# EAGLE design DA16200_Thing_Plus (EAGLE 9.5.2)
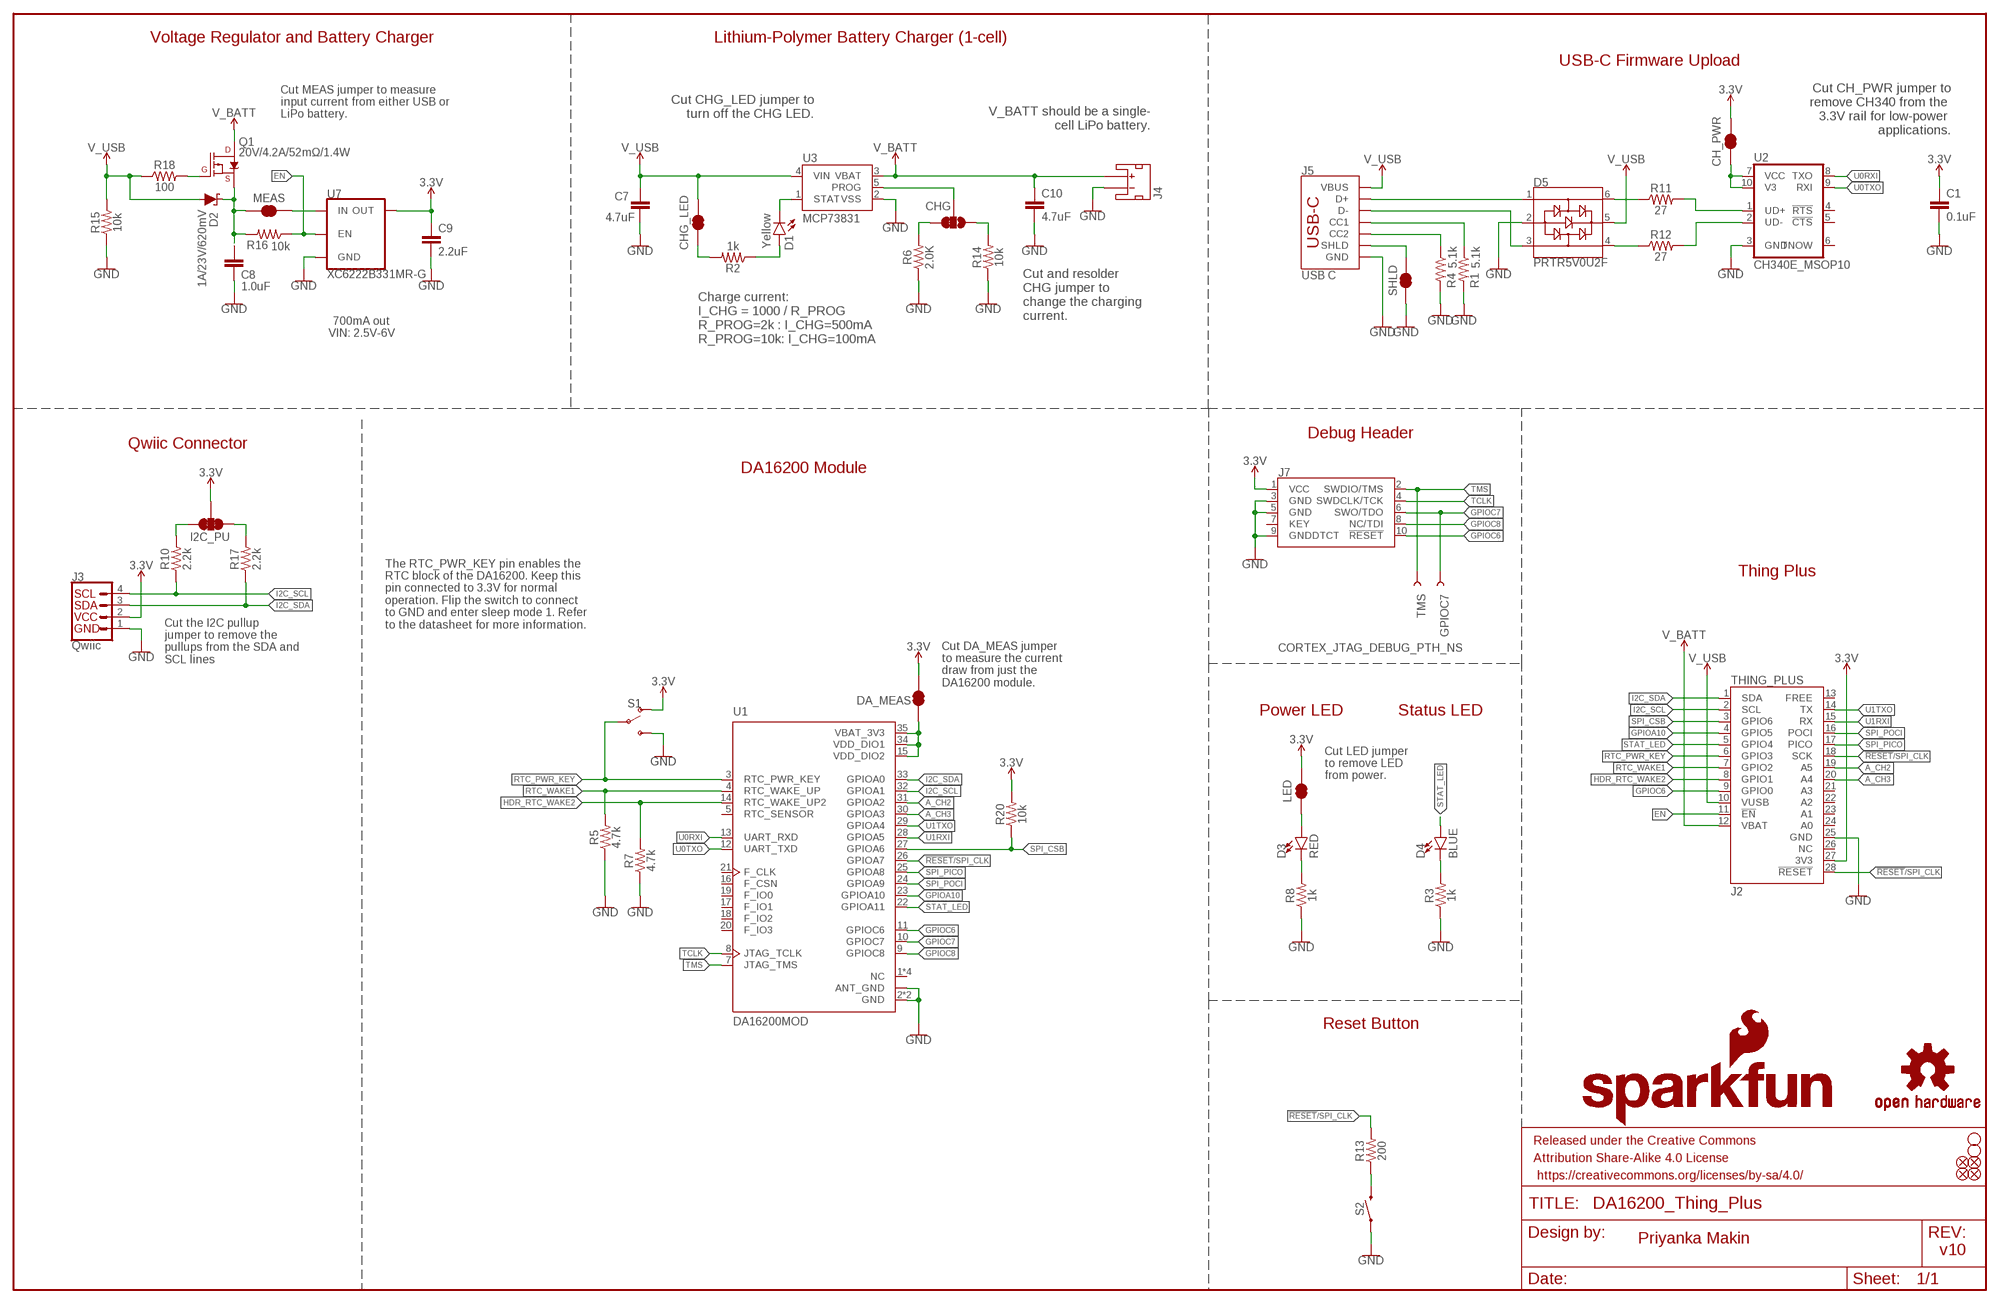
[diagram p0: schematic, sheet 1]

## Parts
C1  0.1uF  0.1UF-0402T-16V-10%  [0402-TIGHT]
C7  4.7uF  4.7UF-0402_TIGHT-6.3V-20%-X5R  [0402-TIGHT]
C8  1.0uF  1.0UF-0402T-16V-10%  [0402-TIGHT]
C9  2.2uF  2.2UF-0402_TIGHT-10V-10%-X5R  [0402-TIGHT]
C10  4.7uF  4.7UF-0402_TIGHT-6.3V-20%-X5R  [0402-TIGHT]
CH_PWR  JUMPER-SMT_2_NC_TRACE_SILK  [SMT-JUMPER_2_NC_TRACE_SILK]
CHG  JUMPER-SMT_3_1-NC_TRACE_SILK  [SMT-JUMPER_3_1-NC_TRACE_SILK]
CHG_LED  JUMPER-SMT_2_NC_TRACE_SILK  [SMT-JUMPER_2_NC_TRACE_SILK]
D1  Yellow  LED-YELLOW0603  [LED-0603]
D2  1A/23V/620mV  DIODE-SCHOTTKY-BAT20J  [SOD-323]
D3  RED  LED-RED0603  [LED-0603]
D4  BLUE  LED-BLUE0603  [LED-0603]
D5  PRTR5V0U2F  [SOT886]
DA_MEAS  JUMPER-SMT_2_NC_TRACE_SILK  [SMT-JUMPER_2_NC_TRACE_SILK]
FD1  FIDUCIALUFIDUCIAL  [FIDUCIAL-MICRO]
FD2  FIDUCIALUFIDUCIAL  [FIDUCIAL-MICRO]
FD3  FIDUCIALUFIDUCIAL  [FIDUCIAL-MICRO]
FD4  FIDUCIALUFIDUCIAL  [FIDUCIAL-MICRO]
FRAME1  FRAME-LEDGER  [CREATIVE_COMMONS]
GPIOC7  TEST-POINT3  [PAD.03X.03]
H3  STAND-OFF  [STAND-OFF]
H4  STAND-OFF  [STAND-OFF]
I2C_PU  JUMPER-SMT_3_2-NC_TRACE_SILK  [SMT-JUMPER_3_2-NC_TRACE_SILK]
J2  THING_PLUS  [THING_PLUS]
J3  Qwiic  QWIIC_CONNECTORJS-1MM  [JST04_1MM_RA]
J4  JST_2MM_MALE  [JST-2-SMD]
J5  USB C  USB_C_4-LAYER-ISOLATED  [USB-C-16P-4LAYER-ISOLATED]
J7  CORTEX_JTAG_DEBUG_PTH_NS  [2X5-PTH-1.27MM-NO_SILK]
LED  JUMPER-SMT_2_NC_TRACE_SILK  [SMT-JUMPER_2_NC_TRACE_SILK]
LOGO1  OSHW-LOGOS  [OSHW-LOGO-S]
LOGO2  SFE_LOGO_NAME_FLAME.1_INCH  [SFE_LOGO_NAME_FLAME_.1]
MEAS  JUMPER-COMBO_2_NC_TRACE  [COMBO-JUMPER_2_NC_TRACE]
Q1  20V/4.2A/52mΩ/1.4W  MOSFET_PCH-DMG2305UX-7  [SOT23-3]
R1  5.1k  5.1KOHM-0402T-1/16W-1%  [0402-TIGHT]
R2  1k  1KOHM-0402T-1/16W-1%  [0402-TIGHT]
R3  1k  1KOHM-0402T-1/16W-1%  [0402-TIGHT]
R4  5.1k  5.1KOHM-0402T-1/16W-1%  [0402-TIGHT]
R5  4.7k  4.7KOHM-0402T-1/16W-1%  [0402-TIGHT]
R6  2.0K  2.0KOHM-0402T-1/16W-1%  [0402-TIGHT]
R7  4.7k  4.7KOHM-0402T-1/16W-1%  [0402-TIGHT]
R8  1k  1KOHM-0402T-1/16W-1%  [0402-TIGHT]
R10  2.2k  2.2KOHM-0402T-1/16W-1%  [0402-TIGHT]
R11  27  27OHM  [0402-TIGHT]
R12  27  27OHM  [0402-TIGHT]
R13  200  200OHM-0402T-1/16W-1%  [0402-TIGHT]
R14  10k  10KOHM-0402T-1/16W-1%  [0402-TIGHT]
R15  10k  10KOHM-0402T-1/16W-1%  [0402-TIGHT]
R16  10k  10KOHM-0402T-1/16W-1%  [0402-TIGHT]
R17  2.2k  2.2KOHM-0402T-1/16W-1%  [0402-TIGHT]
R18  100  100OHM-0402-TIGHT-1/16W-1%  [0402-TIGHT]
R20  10k  10KOHM-0402T-1/16W-1%  [0402-TIGHT]
S1  SWITCH-SPDT-SMD-AYZ0202  [SWITCH_DPDT_SMD_AYZ0202]
S2  MOMENTARY-SWITCH-SPST-SMD-5.2MM-TALL  [TACTILE_SWITCH_SMD_5.2MM]
SHLD  JUMPER-SMT_2_NC_TRACE_SILK  [SMT-JUMPER_2_NC_TRACE_SILK]
TMS  TEST-POINT3  [PAD.03X.03]
U1  DA16200MOD  DA16200MOD-AAC4WA32  [XCVR_DA16200MOD-AAC4WA32]
U2  CH340E_MSOP10  [MSOP10]
U3  MCP73831  [SOT23-5]
U7  XC6222B331MR-G  [SOT23-5]

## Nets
3.3V: C1.1 C9.1 CH_PWR.2 DA_MEAS.2 I2C_PU.2 J2.27(3V3) J3.2 J7.1(VCC) LED.2 R20.2 S1.1(O) U7.5(OUT)
!RESET!/SPI_CLK: J2.18(SCK) J2.28(!RESET) R13.2 U1.26(GPIOA7)
A_CH2: J2.19(A5) U1.31(GPIOA2)
A_CH3: J2.20(A4) U1.30(GPIOA3)
EN: J2.11(!EN) R16.1 U7.3(EN)
GND: C1.2 C7.2 C8.2 C9.2 C10.2 D5.2 J2.25(GND) J3.1 J4.1(-) J5.GND J5.GND2(GND) J7.3(GND) J7.5(GND) J7.9(GNDDTCT) R1.2 R3.1 R4.2 R5.1 R6.1 R7.1 R8.1 R14.1 R15.1 S1.3(S) S2.1 SHLD.1 U1.2(GND) U1.ANT_GND U1.GND U2.3(GND) U3.2(VSS) U7.2(GND)
GPIOA10: J2.4(GPIO5) U1.23(GPIOA10)
GPIOC6: J2.9(GPIO0) J7.10(!RESET) U1.11(GPIOC6)
GPIOC7: GPIOC7.1 J7.6(SWO/TDO) U1.10(GPIOC7)
GPIOC8: J7.8(NC/TDI) U1.9(GPIOC8)
HDR_RTC_WAKE2: J2.8(GPIO1) R7.2 U1.14(RTC_WAKE_UP2)
I2C_SCL: J2.2(SCL) J3.4 R10.1 U1.32(GPIOA1)
I2C_SDA: J2.1(SDA) J3.3 R17.1 U1.33(GPIOA0)
N$1: D4.C R3.2
N$2: I2C_PU.3 R10.2
N$3: I2C_PU.1 R17.2
N$4: D3.A LED.1
N$5: D5.1 J5.A6(D+) J5.B6(D+)
N$6: D5.3 J5.A7(D-) J5.B7(D-)
N$7: D3.C R8.2
N$8: R13.1 S2.3
N$9: D1.C U3.1(STAT)
N$10: CHG.3 R6.2
N$11: J5.A5(CC1) R1.1
N$12: J5.B5(CC2) R4.1
N$13: D5.6 R11.1
N$14: CHG.2 U3.5(PROG)
N$15: C8.1 D2.C MEAS.1 MEAS.3 Q1.2(S) R16.2
N$16: D5.4 R12.1
N$17: D1.A R2.1
N$18: R11.2 U2.1(UD+)
N$19: R12.2 U2.2(UD-)
N$20: CHG.1 R14.2
N$21: Q1.1(G) R18.2
N$22: MEAS.2 MEAS.4 U7.1(IN)
N$23: CHG_LED.1 R2.2
N$24: J5.SHLD1(SHLD) J5.SHLD2(SHLD) J5.SHLD3(SHLD) J5.SHLD4(SHLD) J5.SHLD5(SHLD) J5.SHLD6(SHLD) J5.SHLD7(SHLD) J5.SHLD8(SHLD) SHLD.2
N$25: DA_MEAS.1 U1.15(VDD_DIO2) U1.34(VDD_DIO1) U1.35(VBAT_3V3)
N$26: CH_PWR.1 U2.7(VCC) U2.10(V3)
RTC_PWR_KEY: J2.6(GPIO3) S1.2(P) U1.3(RTC_PWR_KEY)
RTC_WAKE1: J2.7(GPIO2) R5.2 U1.4(RTC_WAKE_UP)
SPI_CSB: J2.3(GPIO6) R20.1 U1.27(GPIOA6)
SPI_PICO: J2.17(PICO) U1.25(GPIOA8)
SPI_POCI: J2.16(POCI) U1.24(GPIOA9)
STAT_LED: D4.A J2.5(GPIO4) U1.22(GPIOA11)
TCLK: J7.4(SWDCLK/TCK) U1.8(JTAG_TCLK)
TMS: J7.2(SWDIO/TMS) TMS.1 U1.7(JTAG_TMS)
U0RXI: U1.13(UART_RXD) U2.8(TXO)
U0TXO: U1.12(UART_TXD) U2.9(RXI)
U1RXI: J2.15(RX) U1.28(GPIOA5)
U1TXO: J2.14(TX) U1.29(GPIOA4)
V_BATT: C10.1 J2.12(VBAT) J4.2(+) Q1.3(D) U3.3(VBAT)
V_USB: C7.1 CHG_LED.2 D2.A D5.5 J2.10(VUSB) J5.VBUS1(VBUS) J5.VBUS2(VBUS) R15.2 R18.1 U3.4(VIN)
Unconnected: J2.13(FREE) J2.21(A3) J2.22(A2) J2.23(A1) J2.24(A0) J2.26(NC) J4.NC1(PAD1) J4.NC2(PAD2) J7.7(KEY) U1.1(NC) U1.5(RTC_SENSOR) U1.6(NC) U1.16(F_CSN) U1.17(F_IO1) U1.18(F_IO2) U1.19(F_IO0) U1.20(F_IO3) U1.21(F_CLK) U1.36(NC) U1.37(NC) U2.4(!RTS) U2.5(!CTS) U2.6(TNOW)

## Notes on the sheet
- Voltage Regulator and Battery Charger | Lithium-Polymer Battery Charger (1-cell)
- USB-C Firmware Upload
- Cut CH_PWR jumper to
  remove CH340 from the 
  3.3V rail for low-power 
  applications.
- Cut CHG_LED jumper to
  turn off the CHG LED.
- V_BATT should be a single-
  cell LiPo battery.
- Cut MEAS jumper to measure
  input current from either USB or 
  LiPo battery.
- Cut and resolder
  CHG jumper to 
  change the charging
  current.
- Charge current:
  I_CHG = 1000 / R_PROG
  R_PROG=2k : I_CHG=500mA
  R_PROG=10k: I_CHG=100mA
- 700mA out
  VIN: 2.5V-6V
- Debug Header
- Qwiic Connector
- DA16200 Module
- Thing Plus
- The RTC_PWR_KEY pin enables the 
  RTC block of the DA16200. Keep this 
  pin connected to 3.3V for normal 
  operation. Flip the switch to connect 
  to GND and enter sleep mode 1. Refer 
  to the datasheet for more information.
- Cut the I2C pullup 
  jumper to remove the 
  pullups from the SDA and 
  SCL lines
- Cut DA_MEAS jumper
  to measure the current
  draw from just the
  DA16200 module.
- Power LED | Status LED
- Cut LED jumper
  to remove LED
  from power.
- Reset Button
- Priyanka Makin
- v10

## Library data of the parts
C1 = SparkFun-Capacitors:0.1UF: 0.1µF ceramic capacitors; PROD_ID: CAP-12416
C7 C10 = SparkFun-Capacitors:4.7UF: 4.7µF ceramic capacitors; PROD_ID: CAP-14240
C8 = SparkFun-Capacitors:1.0UF: 1µF ceramic capacitors; PROD_ID: CAP-12417
C9 = SparkFun-Capacitors:2.2UF: 2.2µF ceramic capacitors; PROD_ID: CAP-14232
CH_PWR CHG_LED DA_MEAS LED SHLD = SparkFun-Jumpers:JUMPER-SMT_2_NC_TRACE: Normally closed trace jumper
CHG = SparkFun-Jumpers:JUMPER-SMT_3_1-NC_TRACE: Normally closed trace jumper (1 of 2 connections) This jumper has a trace between two pads so it's normally closed (NC). The other connection is normally open (NO). Use a razor knife to open the connection. For best results follow the IPC guidelines for cutting traces: Cutout at least 0.063 mm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
D1 = SparkFun-LED:LED-YELLOW: Yellow SMD LED; PROD_ID: DIO-09003
D2 = SparkFun-DiscreteSemi:DIODE-SCHOTTKY: Schottky diode; PROD_ID: DIO-11623
D3 = SparkFun-LED:LED-RED: Red SMD LED; PROD_ID: DIO-00819
D4 = SparkFun-LED:LED-BLUE: Blue SMD LED; PROD_ID: DIO-08575
D5 = SparkFun-IC-Power:PRTR5V0U2: A small ESD protection device. Most commonly used on USB D+/D- signals to protect large, expensive, or especially sensitive USB enabled devices.; PROD_ID: DIO-14084
FD1-FD4 = SparkFun-Aesthetics:FIDUCIAL: Fiducial Alignment Points
FRAME1 = SparkFun-Aesthetics:FRAME-LEDGER: Schematic Frame - Ledger
GPIOC7 TMS = SparkFun-Connectors:TEST-POINT: SparkFun Test Points
H3 H4 = SparkFun-Hardware:STAND-OFF: Stand Off
I2C_PU = SparkFun-Jumpers:JUMPER-SMT_3_2-NC_TRACE: Normally closed trace jumper (2 of 2 connections) This jumper has a trace between all three pads so they are normally closed (NC). Use a razor knife to open the connection(s). For best results follow the IPC guidelines for cutting traces: Cutout at least 0.063 mm (0.005 in). Remove all loose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
J2 = SparkFun-Boards:THING_PLUS
J3 = SparkFun-Connectors:QWIIC_CONNECTOR: SparkFun I2C Standard Qwiic Connector An SMD 1mm pitch JST connector makes it easy and quick (get it? Qwiic?) to connect I2C devices to each other. The Qwiic system enables fast and solderless connection between popular platforms and various sensors and actuators. We carry 200mm, 100mm, 50mm, and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; PROD_ID: CONN-13694; VALUE: QWIIC_RIGHT_ANGLE
J4 = SparkFun-Connectors:JST_2MM_MALE: JST 2MM MALE RA CONNECTOR Two pin, compact surface mount connector. Commonly used as a battery input connection point. We really like the solid locking feeling and high current rating on these small connectors. We use these all the time as battery connectors. Mates to single-cell LiPo batteries.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; PROD_ID: CONN-11443; SF_ID: PRT-08612
J5 = SparkFun-Connectors:USB_C: USB Type C 16Pin Connector Super Speed pins not available on the 16-pin purely SMD connector so this part is best for USB 2.0 implementations. D1 and D2 are tied together enabling D+/- no matter which way the cable is plugged into the connector. The two channel configuration pins (CC1/2) are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; PROD_ID: CONN-14122; VALUE: USB Female Type C Connector
J7 = SparkFun-Connectors:CORTEX_JTAG_DEBUG: Cortex Debug Connector - 10 pin Supports JTAG debug, Serial Wire debug, and Serial Wire Viewer. PTH and SMD connector options available. General Connector Information Products: PTH Connector -via Digi-Key SparkFun PSoc SparkFun T
LOGO1 = SparkFun-Aesthetics:OSHW-LOGO: Open-Source Hardware (OSHW) Logo
LOGO2 = SparkFun-Aesthetics:SFE_LOGO_NAME_FLAME: SparkFun Font Logo w/ Flame
MEAS = SparkFun-Jumpers:JUMPER-COMBO_2_NC_TRACE
Q1 = SparkFun-DiscreteSemi:MOSFET_PCH: P-channel MOSFETs Voltage controlled devices that allow control of high current outputs. SparkFun Products: SparkFun ESP32 Thing SparkFun ESP8266 Thing SparkFun Pi Servo HAT V2 DMG2305UX-7 (20V/4.2A/SOT23-3); PROD_ID: TRANS-14388
R1 R4 = SparkFun-Resistors:5.1KOHM; PROD_ID: RES-14340
R2 R3 R8 = SparkFun-Resistors:1KOHM: 1kΩ resistor; PROD_ID: RES-14342
R5 R7 = SparkFun-Resistors:4.7KOHM: 4.7kΩ resistor; PROD_ID: RES-15343
R6 = SparkFun-Resistors:2.0KOHM: 2kΩ resistor; PROD_ID: RES-15406
R10 R17 = SparkFun-Resistors:2.2KOHM: 2.2kΩ resistor; PROD_ID: RES-14341
R11 R12 = SparkFun-Resistors:27OHM: 27Ω resistor; PROD_ID: RES-15238
R13 = SparkFun-Resistors:200OHM: 200Ω resistor; PROD_ID: RES-15550
R14-R16 R20 = SparkFun-Resistors:10KOHM: 10kΩ resistor; PROD_ID: RES-14241
R18 = SparkFun-Resistors:100OHM: 100Ω resistor; PROD_ID: RES-14962
S1 = SparkFun-Switches:SWITCH-SPDT: Single Pole, Double Throw (SPDT) Switch Single-pole, double-throw (SPDT) switch. Variant Overview SMD-AYZ0202 Surface Mount DPDT Switch (COM-00597) Used on e.g. LilyPad Arduino USB - ATmega32U4 Board PTH-11.6X4.0MM SPDT Mini Power Switch (COM-00102) Used on e.g. SparkFun Simon Says - Through-Hole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; PROD_ID: SWCH-08179; SF_ID: COM-00597
S2 = SparkFun-Switches:MOMENTARY-SWITCH-SPST: Momentary Switch (Pushbutton) - SPST; PROD_ID: SWCH-14139
U1 = SparkFun-RF:DA16200MOD-AAC4WA32: Check prices; PROD_ID: IC-16179
U2 = SparkFun-IC-Comms:CH340E; PROD_ID: IC-14135
U3 = SparkFun-IC-Power:MCP73831: MCP73831T Li-Ion, Li-Pol Controller Miniature single cell, fully integrated Li-Ion, Li-polymer charge management controller Datasheet SparkFun Products: SparkFun ESP32 Thing SparkFun 9DoF Razor IMU M0; PROD_ID: IC-09995
U7 = SparkFun-IC-Power:XC6222; IOUT: 700mA; PROD_ID: VREG-16775; VOUT: 3.3V

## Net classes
0 default: width 0 mm, drill 0 mm
2 Clock: width 0.089 mm, clearance 0.178 mm

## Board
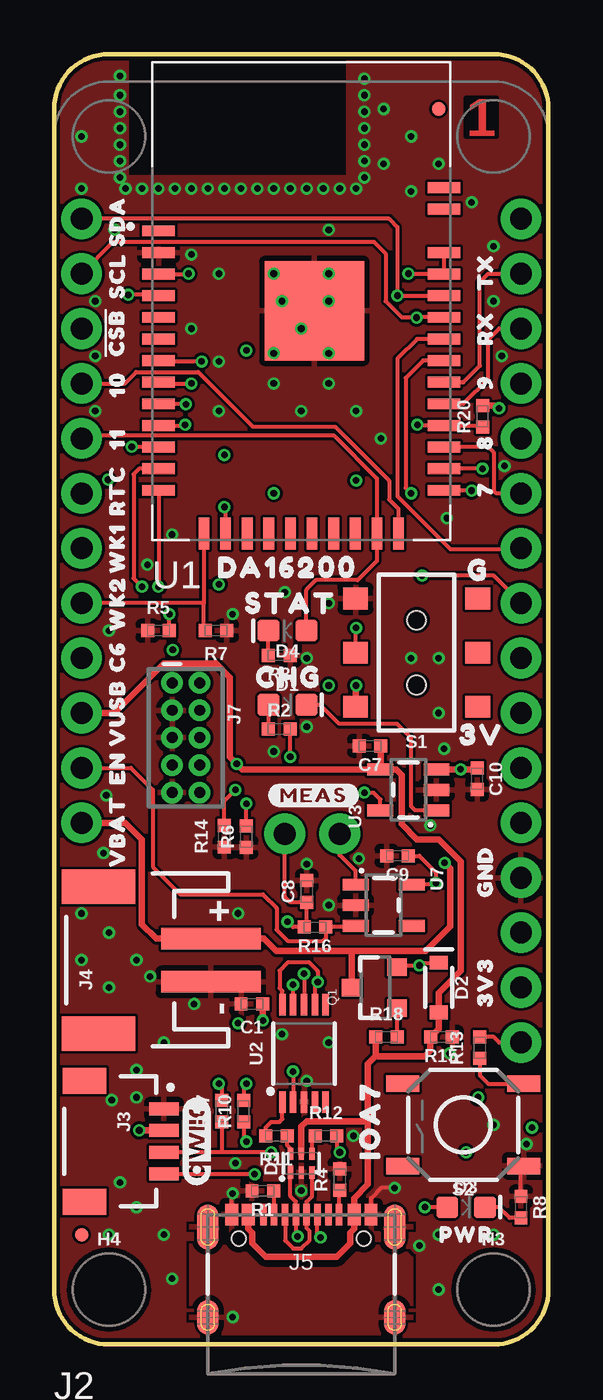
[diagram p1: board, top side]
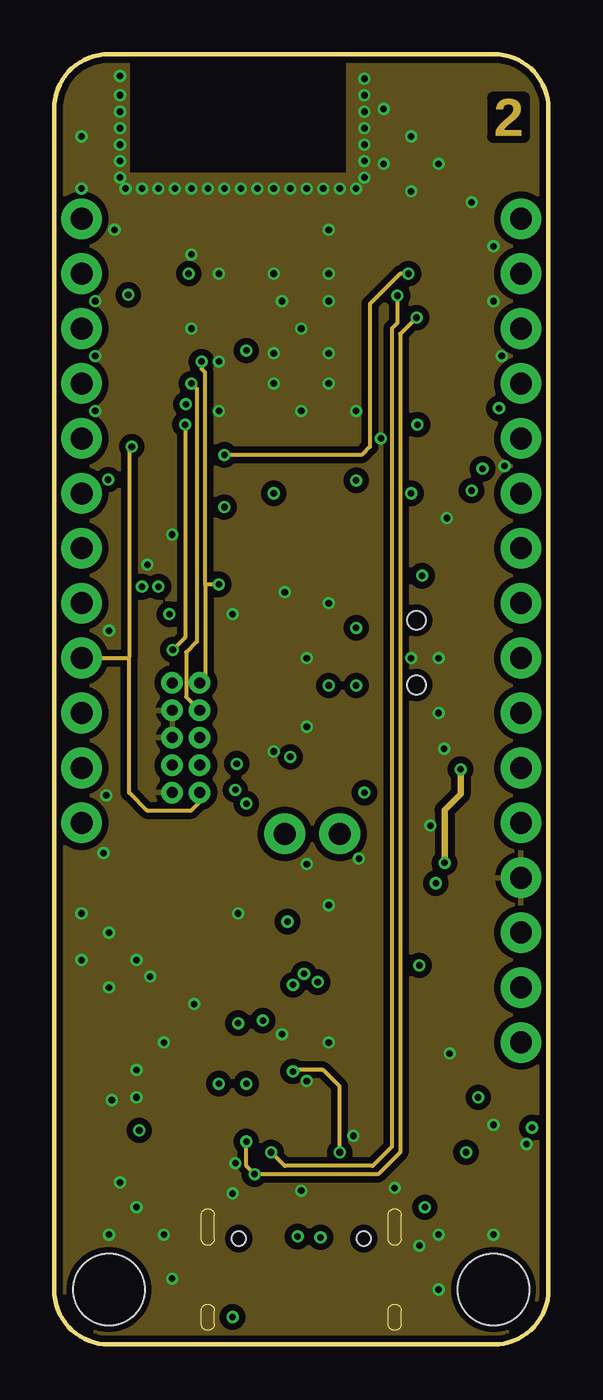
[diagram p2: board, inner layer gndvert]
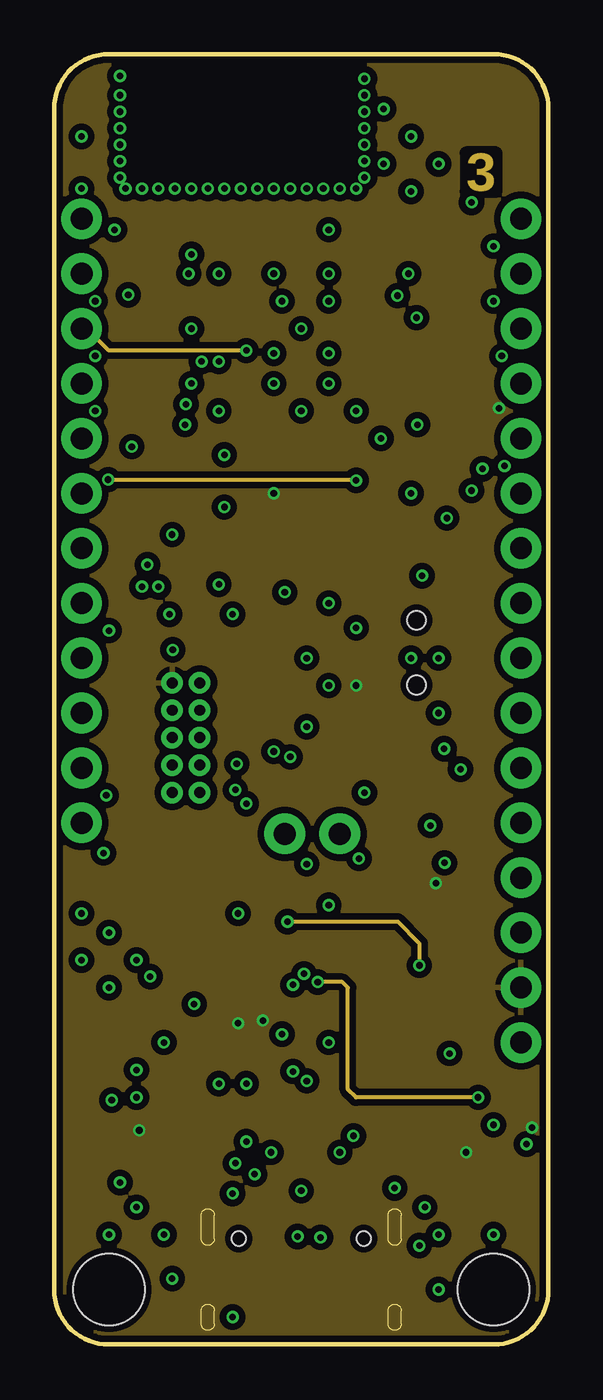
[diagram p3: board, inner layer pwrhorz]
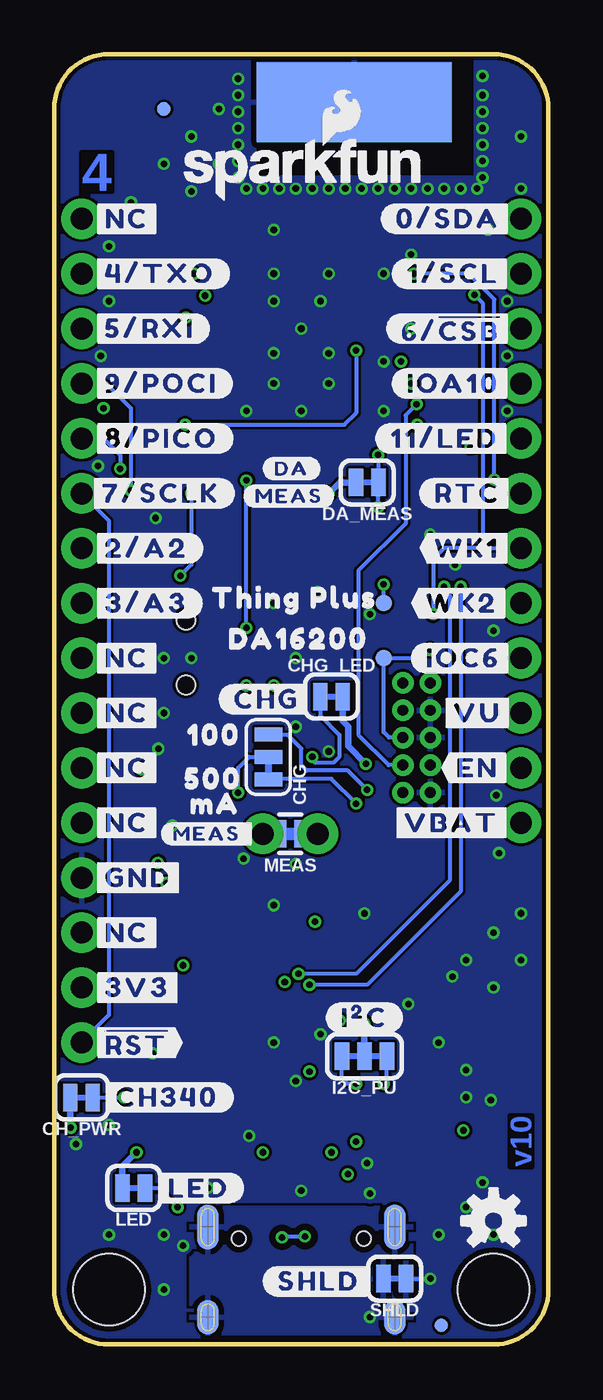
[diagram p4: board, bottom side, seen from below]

Size 22.86 x 59.69 mm. Coordinates in mm from the lower left corner, seen from the top.
Outline: 2.54,59.69 20.32,59.69 arc-90 22.86,57.15 22.86,2.54 arc-90 20.32,0 2.54,0 arc-90 0,2.54 0,57.15 arc-90 2.54,59.69
Copper layers (1*2*15*16): Top 0.035559375mm / dielectric 0.47751875mm / gndvert 0.035559375mm / dielectric 0.47751875mm / pwrhorz 0.035559375mm / dielectric 0.47751875mm / Bottom 0.035559375mm
Design rules "SparkFun-4-Layer-Minimum-JLCPCB": minimum track width 5mil, minimum drill 0.2mm, track to track 5mil, track to pad 5mil, pad to pad 5mil, via to via 5mil, smd to smd 5mil, copper to edge 7mil, drill to drill 7mil, minimum pad ring 5mil, minimum via ring 5mil, stop-mask expansion 2.5mil, vias tented up to drill 25mil, thermal gap 10mil

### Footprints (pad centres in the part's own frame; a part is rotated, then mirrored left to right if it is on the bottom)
0402-TIGHT = smd 0.6 x 0.6: 1 -0.5,0; 2 0.5,0
SMT-JUMPER_2_NC_TRACE_SILK = smd 0.66 x 1.27: 1 -0.521,0; 2 0.521,0
SMT-JUMPER_3_1-NC_TRACE_SILK = smd 0.66 x 1.27: 1 -1.041,0; 2 0,0; 3 1.041,0
LED-0603 = smd 1 x 1: A -0.877,0; C 0.877,0
SOD-323 = smd 0.63 x 0.83: A 1.15,0; C -1.15,0
SOT886 = smd 0.61 x 0.25: 1 -0.405,0.5 | smd 0.56 x 0.25: 2 -0.43,0; 3 -0.43,-0.5; 4 0.43,-0.5; 5 0.43,0; 6 0.43,0.5
FIDUCIAL-MICRO = smd 0.635 x 0.635: 1 0,0
PAD.03X.03 = smd 0.762 x 0.762: 1 0,0
STAND-OFF = hole 3.302: 0,0
SMT-JUMPER_3_2-NC_TRACE_SILK = smd 0.66 x 1.27: 1 -1.041,0; 2 0,0; 3 1.041,0
THING_PLUS = drill 1.016 pad 1.88: 1 1.27,52.07; 2 1.27,49.53; 3 1.27,46.99; 4 1.27,44.45; 5 1.27,41.91; 6 1.27,39.37; 7 1.27,36.83; 8 1.27,34.29; 9 1.27,31.75; 10 1.27,29.21; 11 1.27,26.67; 12 1.27,24.13; 13 21.59,52.07; 14 21.59,49.53; 15 21.59,46.99; 16 21.59,44.45; 17 21.59,41.91; 18 21.59,39.37; 19 21.59,36.83; 20 21.59,34.29; 21 21.59,31.75; 22 21.59,29.21; 23 21.59,26.67; 24 21.59,24.13; 25 21.59,21.59; 26 21.59,19.05; 27 21.59,16.51; 28 21.59,13.97
JST04_1MM_RA = smd 0.6 x 1.35: 1 -1.5,0; 2 -0.5,0; 3 0.5,0; 4 1.5,0 | smd 1.2 x 2: NC1 2.8,-3.675; NC2 -2.8,-3.675
JST-2-SMD = smd 1 x 4.6: 1 -1,-3.7; 2 1,-3.7 | smd 1.6 x 3.4: NC1 -3.4,1.5; NC2 3.4,1.5
USB-C-16P-4LAYER-ISOLATED = smd 0.3 x 1: A5 -1.25,-0.34; A6 -0.25,-0.34; A7 0.25,-0.34; A8 1.25,-0.34; B5 1.75,-0.34; B6 0.75,-0.34; B7 -0.75,-0.34; B8 -1.75,-0.34 | smd 0.6 x 1: GND -3.225,-0.34; GND2 3.225,-0.34; VBUS1 -2.45,-0.34; VBUS2 2.45,-0.34 | smd 1 x 2.1: SHLD1 -4.32,-0.915; SHLD2 4.32,-0.915 | smd 1 x 2.1 bottom: SHLD3 -4.32,-0.915; SHLD4 4.32,-0.915 | smd 1 x 1.6: SHLD5 -4.32,-5.095; SHLD8 4.32,-5.095 | smd 1 x 1.6 bottom: SHLD6 -4.32,-5.095; SHLD7 4.32,-5.095 | hole 0.65: -2.89,-1.445; 2.89,-1.445
2X5-PTH-1.27MM-NO_SILK = drill 0.508 pad 1: 1 -2.54,-0.635; 2 -2.54,0.635; 3 -1.27,-0.635; 4 -1.27,0.635; 5 0,-0.635; 6 0,0.635; 7 1.27,-0.635; 8 1.27,0.635; 9 2.54,-0.635; 10 2.54,0.635
COMBO-JUMPER_2_NC_TRACE = smd 0.635 x 1.27: 1 -0.508,0; 2 0.508,0 | drill 1.016 pad 1.88: 3 -1.27,0; 4 1.27,0
SOT23-3 = smd 0.8 x 0.9: 1 -0.95,-1; 2 0.95,-1; 3 0,1.1
SWITCH_DPDT_SMD_AYZ0202 = smd 1 x 1.15: 1 -2.5,2.825; 2 0,2.825; 3 2.5,2.825; 4 -2.5,-2.825; 5 0,-2.825; 6 2.5,-2.825 | hole 0.85: 1.5,0; -1.5,0
TACTILE_SWITCH_SMD_5.2MM = smd 1.524 x 0.762: 1 -2.794,1.905; 2 2.794,1.905; 3 -2.794,-1.905; 4 2.794,-1.905
XCVR_DA16200MOD-AAC4WA32 = smd 1.5 x 0.5: 1 -6.6,3.25; 2 -6.6,2.25; 3 -6.6,1.25; 4 -6.6,0.25; 5 -6.6,-0.75; 6 -6.6,-1.75; 7 -6.6,-2.75; 8 -6.6,-3.75; 9 -6.6,-4.75; 10 -6.6,-5.75; 11 -6.6,-6.75; 12 -6.6,-7.75; 13 -6.6,-8.75; 24 6.6,-8.75; 25 6.6,-7.75; 26 6.6,-6.75; 27 6.6,-5.75; 28 6.6,-4.75; 29 6.6,-3.75; 30 6.6,-2.75; 31 6.6,-1.75; 32 6.6,-0.75; 33 6.6,0.25; 34 6.6,1.25; 35 6.6,2.25; 36 6.6,4.25; 37 6.6,5.25 | smd 0.5 x 1.5: 14 -4.5,-10.75; 15 -3.5,-10.75; 16 -2.5,-10.75; 17 -1.5,-10.75; 18 -0.5,-10.75; 19 0.5,-10.75; 20 1.5,-10.75; 21 2.5,-10.75; 22 3.5,-10.75; 23 4.5,-10.75 | smd 9 x 3.7 bottom: ANT_GND -2.45,9.2 | smd 4.6 x 4.6: GND 0.61,-0.45
MSOP10 = smd 1 x 0.3: 1 -2.25,1; 2 -2.25,0.5; 3 -2.25,0; 4 -2.25,-0.5; 5 -2.25,-1; 6 2.25,-1; 7 2.25,-0.5; 8 2.25,0; 9 2.25,0.5; 10 2.25,1
SOT23-5 = smd 0.55 x 1.2: 1 -0.95,-1.3; 2 0,-1.3; 3 0.95,-1.3; 4 0.95,1.3; 5 -0.95,1.3

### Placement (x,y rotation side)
C1  9.14,15.75 180 top
C7  14.61,27.69 180 top
C8  11.68,20.95 90 top
C9  15.88,22.61 180 top
C10  19.56,26.16 270 top
CH_PWR  21.59,11.43 180 bottom
CHG  12.95,27.18 270 bottom
CHG_LED  10.03,29.97 0 bottom
D1  10.79,29.59 0 top
D2  17.78,16.51 270 top
D3  19.05,6.35 0 top
D4  10.79,33.02 180 top
D5  11.43,8.38 90 top
DA_MEAS  8.38,39.88 180 bottom
FD1  1.27,5.08 0 top
FD2  17.78,57.15 0 top
FD3  4.95,0.89 0 bottom
FD4  17.78,57.15 0 bottom
FRAME1  not placed on the board
GPIOC7  7.62,31.75 0 bottom
H3  20.32,2.54 0 top
H4  2.54,2.54 0 top
I2C_PU  8.51,13.34 180 bottom
J2  0,0 0 top
J3  5.08,9.4 270 top
J4  3.56,17.78 90 top
J5  11.43,6.35 0 top
J7  6.1,28.07 270 top
LED  19.18,7.24 180 bottom
LOGO1  2.54,5.71 0 bottom
LOGO2  11.3,54.36 0 bottom
MEAS  11.94,23.62 180 bottom
Q1  14.86,16.51 90 top
R1  9.65,7.11 180 top
R2  10.41,28.47 0 top
R3  10.41,31.88 180 top
R4  13.21,7.62 90 top
R5  4.83,33.02 0 top
R6  8.89,23.5 90 top
R7  7.49,33.02 180 top
R8  21.59,6.35 270 top
R10  8.76,10.79 90 top
R11  10.28,9.65 180 top
R12  12.58,9.65 0 top
R13  19.68,13.72 90 top
R14  7.87,23.5 90 top
R15  17.91,14.22 180 top
R16  12.06,19.3 180 top
R17  7.75,10.79 90 top
R18  15.38,14.22 0 top
R20  19.81,42.93 90 top
S1  16.76,32 90 top
S2  18.92,10.16 180 top
SHLD  7.11,3.05 180 bottom
TMS  7.62,34.29 0 bottom
U1  11.43,48.26 0 top
U2  11.56,13.46 90 top
U3  16.38,25.65 90 top
U7  15.24,20.32 270 top
U$1  [STAT0]  8.13,34.29 0 top
U$2  [CHG0]  8.64,30.86 0 top
U$3  [#MEAS_#0]  17.91,23.62 0 bottom
U$4  [G0]  18.41,35.81 0 top
U$5  [##RST##0]  21.21,13.97 0 bottom
U$6  [#VU#0]  5.08,29.21 0 bottom
U$7  [#IOA10#0]  7.24,44.45 0 bottom
U$8  [#MEAS#0]  9.91,25.4 0 top
U$9  [3V0]  18.03,28.19 0 top
U$10  [#CH340#0]  20.7,11.43 0 bottom
U$11  [#0#SDA#0]  7.75,52.07 0 bottom
U$12  [#1#SCL#0]  7.24,49.53 0 bottom
U$13  [IOA7_0]  14.61,7.87 90 top
U$14  [#NC#0]  21.21,31.75 0 bottom
U$15  [#NC#0]  21.21,29.21 0 bottom
U$16  [PWR0]  19.05,5.08 0 top
U$17  [#DA#0]  13.21,40.51 0 bottom
U$18  [#NC#0]  21.21,26.67 0 bottom
U$19  [#NC#0]  21.21,24.13 0 bottom
U$20  [#NC#0]  21.21,19.05 0 bottom
U$21  [5000]  17.53,26.16 0 bottom
U$22  [1000]  17.4,28.19 0 bottom
U$23  [MA0]  17.27,25.02 0 bottom
U$24  [SDA0]  2.92,50.29 90 top
U$25  [SCL0]  2.92,47.88 90 top
U$26  [#CSB#0]  2.79,45.21 90 top
U$27  [#4#TXO#0]  21.21,49.53 0 bottom
U$28  [110]  2.92,40.89 90 top
U$29  [#MEAS#0]  14.1,39.24 0 bottom
U$30  [#VBAT#0]  7.37,24.13 0 bottom
U$31  [ORDERING_INSTRUCTIONS]  not placed on the board
U$32  [100]  2.92,43.31 90 top
U$33  [RTC0]  2.92,37.85 90 top
U$34  [WK10]  2.92,35.18 90 top
U$35  [WK20]  2.92,32.51 90 top
U$36  [#5#RXI#0]  21.21,46.99 0 bottom
U$37  [EN0]  2.92,25.4 90 top
U$38  [VUSB0]  2.92,27.18 90 top
U$39  [VBAT0]  2.92,21.59 90 top
U$40  [#NC#0]  21.21,52.07 0 bottom
U$41  [TX0]  19.94,48.26 90 top
U$42  [RX0]  19.94,45.72 90 top
U$44  [90]  19.94,43.69 90 top
U$45  [80]  19.94,40.89 90 top
U$47  [70]  19.94,38.73 90 top
U$50  [#GND#0]  21.21,21.59 0 bottom
U$51  [#3V3#0]  21.21,16.51 0 bottom
U$53  [#EN#0]  4.95,26.67 0 bottom
U$55  [GND0]  19.94,20.19 90 top
U$56  [THING_PLUS0]  16.26,34.54 0 bottom
U$57  [3V30]  19.94,15.11 90 top
U$59  [#CHG#0]  15.24,29.84 0 bottom
U$60  [#IOC6#0]  6.35,31.75 0 bottom
U$62  [#6##CSB##0]  7.49,46.99 0 bottom
U$63  [#11#LED#0]  8,41.91 0 bottom
U$64  [QWIIC_4MM]  6.6,9.4 90 top
U$65  [C60]  2.92,30.61 90 top
U$66  [#9#POCI#0]  21.21,44.45 0 bottom
U$67  [#8#PICO#0]  21.21,41.91 0 bottom
U$68  [#7#SCLK#0]  21.34,39.37 0 bottom
U$69  [#2#A2#0]  21.21,36.83 0 bottom
U$70  [#3#A3#0]  21.21,34.29 0 bottom
U$71  [#WK2#0]  6.35,34.29 0 bottom
U$72  [#WK1#0]  5.97,36.83 0 bottom
U$73  [#RTC#0]  5.97,39.37 0 bottom
U$80  [DA162000]  15.49,32.64 0 bottom
U$81  [DA162000]  6.86,35.94 0 top
U$82  [#I�C#0]  10.29,15.11 0 bottom
U$84  [#LED#0]  18.29,7.24 0 bottom
U$85  [#SHLD#0]  13.21,2.92 0 bottom

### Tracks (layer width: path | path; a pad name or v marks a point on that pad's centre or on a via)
3.3V  (via drill 0.3)
  Top 0.178: C9.1 16.89,22.61 17.65,21.84 v17.65,21.34 17.65,21.27 U7.5
  Top 0.305: C1.1 9.65,15.74 v9.65,14.99 | J3.2 3.94,9.9 v3.94,9.91 | S1.1 13.94,30.45 v13.97,30.48 | R20.2 20.45,43.43 v20.57,43.31
  Bottom 0.305: LED.2 19.7,8.24 v19.05,8.89 | DA_MEAS.2 9.65,39.88 v10.16,39.37 | CH_PWR.2 22.11,10.05 v22.1,10.03 | I2C_PU.2 v8.51,14.86
  pour pwrhorz (isolate 0.305): 0,0 22.86,0 22.86,59.69 13.59,59.69 13.59,54.1 3.3,54.1 3.3,59.69 0,59.69
!RESET!/SPI_CLK
  Top 0.178: J2.18 20.45,39.37 20.32,39.5 20.32,41.27 20.09,41.51 U1.26 | J2.28 20.57,13.97 20.32,14.22 R13.2
  Bottom 0.178: J2.18 20.32,38.1 20.32,15.24 J2.28
A_CH2
  Top 0.178: U1.31 16.79,46.51 15.88,45.59 15.88,39.24 18.33,36.79 21.55,36.79 J2.19
A_CH3  (via drill 0.3)
  Top 0.178: U1.30 17.06,45.51 16.26,44.7 16.26,39.62 v16.51,39.37 | J2.20 20.32,35.56 v17.02,35.56
  Bottom 0.178: v16.51,39.37 16.51,36.07 v17.02,35.56
EN
  Top 0.178: U7.3 13.87,19.3 R16.1 12.56,18.79 12.45,18.67 10.79,18.67 10.29,19.18 10.29,20.19 9.65,20.83 5.84,20.83 4.57,22.1 4.57,25.65 3.56,26.67 J2.11
GND  (via drill 0.3)
  Top 0.178: R8.1 21.59,8.13 S2.1 | J5.GND 8.21,6.93 v8.26,6.99 | J5.GND2 14.65,6.77 15.12,7.24 v15.75,7.24
  Bottom 0.178: SHLD.1 v5.46,3.05
  other vias: 6.35,50.42 10.54,48.26 11.43,46.99 12.7,48.26 12.7,45.85 10.16,45.85 8.26,33.78 10.67,34.8 11.68,28.57 18.03,27.56 6.48,15.75 4.45,17.02 11.68,22.23 14.1,22.48 3.81,11.43 12.7,20.32 13.84,9.65 11.43,7.11 11.68,12.19 18.29,13.46 16.89,4.57 3.05,57.78 3.05,57.02 3.05,56.26 3.05,55.5 3.05,54.74 3.05,53.98 3.05,58.67 3.3,53.47 4.06,53.47 4.83,53.47 5.59,53.47 6.35,53.47 7.11,53.47 7.87,53.47 8.64,53.47 9.4,53.47 10.16,53.47 10.92,53.47 11.68,53.47 12.45,53.47 13.21,53.47 13.97,53.47 14.35,58.55 14.35,53.98 14.35,54.74 14.35,55.5 14.35,56.26 14.35,57.02 14.35,57.78 1.27,55.88 1.27,53.47 15.24,57.15 16.51,55.88 15.24,54.61 17.78,54.61 16.51,53.34 19.3,52.83 20.32,50.8 12.7,49.53 10.16,49.53 7.62,49.53 7.62,45.47 7.62,43.18 13.97,43.18 15.11,41.91 5.46,37.47 11.68,31.75 12.7,34.29 17.78,31.75 16.51,31.75 17.78,29.21 17.4,24 1.27,19.94 2.54,19.05 3.81,17.78 1.27,17.78 2.54,16.51 3.81,12.7 2.67,11.3 3.05,7.49 3.81,6.35 2.54,5.08 5.08,5.08 17.78,2.54 17.78,5.08 20.32,5.08 21.84,9.27 20.32,10.16 12.7,13.97 10.54,14.35 5.08,13.97 11.43,43.18 12.7,44.45 10.16,44.45 2.54,33.02 6.35,46.99 10.16,27.43 2.79,51.56 1.91,48.26 1.91,45.72 1.91,43.18 12.7,51.56 20.32,48.26 20.7,45.72 20.83,40.64 4.32,36.07 2.41,25.4 2.29,22.73 8.51,19.94 8.38,8.38 18.16,38.23
  pour Bottom (rank 2): 0,59.69 22.86,59.69 22.86,0 0,0
  pour Top (rank 2): 0,59.69 22.86,59.69 22.86,0 0,0
  pour gndvert (isolate 0.305): 0,0 22.86,0 22.86,59.69 13.59,59.69 13.59,54.1 3.43,54.1 3.43,59.69 0,59.69
GPIOA10
  Top 0.178: U1.23 15.93,38.65 15.5,39.09 15.5,39.96 13,42.46 9.19,42.46 6.66,44.98 3.8,44.98 3.26,44.45 J2.4
GPIOC6  (via drill 0.3)
  Top 0.178: U1.11 3.61,41.51 v3.59,41.53
  gndvert 0.178: J2.9 3.43,31.75 3.47,31.79 | v3.59,41.53 3.47,41.4 3.47,31.79 | J7.10 6.73,25.09 6.35,24.71 4.29,24.71 3.47,25.53 3.47,31.79
GPIOC7  (via drill 0.3)
  Top 0.178: v6.06,42.55 6.02,42.51 U1.10
  gndvert 0.178: v6.06,42.55 6.06,32.7 v5.49,32.13
  Bottom 0.178: J7.6 7.37,28.07 7.62,28.32 GPIOC7.1 6.22,31.75 5.84,32.13 v5.49,32.13
GPIOC8  (via drill 0.3)
  Top 0.178: v6.1,43.49 4.85,43.49 U1.9
  Bottom 0.178: v6.1,43.49 6.6,42.98 6.6,37.97 8.79,35.79 8.79,28.19 7.39,26.8 J7.8
HDR_RTC_WAKE2
  Top 0.178: U1.14 6.93,34.29 | 6.93,34.29 J2.8 | R7.2 6.93,32.96 6.93,34.29
I2C_SCL  (via drill 0.3)
  Top 0.178: U1.32 16.78,47.51 v16.76,47.5 16.09,47.5 15.33,48.26 15.33,50.46 14.78,51 2.74,51 J2.2 | v9.27,7.87 5.1,7.87 J3.4 | R10.1 8.76,9.51 v8.89,9.38
  gndvert 0.178: v16.76,47.5 16,46.74 16,8.89 14.99,7.87 v9.27,7.87 8.89,8.26 v8.89,9.38
I2C_SDA  (via drill 0.3)
  Top 0.178: U1.33 v15.88,48.51 15.88,51.69 15.49,52.07 J2.1 | v10.03,8.89 7.75,8.89 | 7.75,8.89 J3.3 | R17.1 7.75,8.89
  gndvert 0.178: v15.88,48.51 15.88,47.24 15.62,46.99 15.62,9.14 14.73,8.26 10.67,8.26 v10.03,8.89
N$1
  Top 0.178: R3.2 D4.C
N$2  (via drill 0.3)
  Top 0.178: v8.89,12.06 8.76,11.94 R10.2
  Bottom 0.178: v8.89,12.06 9.27,12.06 9.55,12.34 I2C_PU.3
N$3  (via drill 0.3)
  Top 0.178: v7.62,12.06 7.75,11.94 R17.2
  Bottom 0.178: v7.62,12.06 7.47,12.22 I2C_PU.1
N$4  (via drill 0.3)
  Top 0.178: D3.A v17.14,6.35
  Bottom 0.178: LED.1 18.03,7.24 v17.14,6.35
N$5  (via drill 0.3)
  Top 0.178: v11.26,5 11.18,5.08 J5.A6 11.18,6.6 10.92,6.86 D5.1 | v12.32,4.95 12.18,5.09 J5.B6
  Bottom 0.178: v12.32,4.95 12.28,5 v11.26,5
N$6
  Top 0.178: J5.B7 10.68,4.81 11.05,4.45 11.43,4.45 11.81,4.83 11.81,5.24 11.68,5.38 J5.A7 11.68,6.6 11.94,6.86 D5.3
N$7
  Top 0.178: R8.2 21.06,5.85 20.56,6.35 D3.C
N$8
  Top 0.178: R13.1 19.68,12.45 20.07,12.06 S2.3
N$9
  Top 0.178: U3.1 16.7,24.7 16.5,24.9 16.5,28.07 15.86,28.7 13.2,28.7 12.31,29.59 D1.C
N$10  (via drill 0.3)
  Top 0.178: R6.2 v8.89,25.02
  Bottom 0.178: CHG.3 12.93,26.16 10.03,26.16 v8.89,25.02
N$11
  Top 0.178: J5.A5 10.18,7.11 R1.1
N$12
  Top 0.178: J5.B5 13.18,7.09 R4.1
N$13
  Top 0.178: D5.6 10.93,9.07 10.78,9.22 R11.1
N$14  (via drill 0.3)
  Top 0.178: v14.35,25.53 14.77,25.53 15.08,25.21 U3.5
  Bottom 0.178: v14.35,25.53 14.35,26.67 13.84,27.18 CHG.2
N$15  (via drill 0.3)
  Top 0.178: Q1.2 15.93,17.53 v16.89,17.53 17.02,17.66 D2.C | v10.79,19.56 10.8,19.56 11.06,19.3 R16.2 11.68,19.42 C8.1 10.92,20.45 10.67,20.71 MEAS.3
  pwrhorz 0.178: v10.79,19.56 15.88,19.56 16.89,18.55 v16.89,17.53
  Bottom 0.178: MEAS.1 MEAS.3
N$16
  Top 0.178: D5.4 11.93,9.65 R12.1
N$17
  Top 0.178: D1.A R2.1
N$18
  Top 0.178: R11.2 9.78,10.03 10.03,10.29 10.41,10.29 10.56,10.43 U2.1
N$19  (via drill 0.3)
  Top 0.178: R12.2 13.08,9.02 v13.21,8.89 | v11.05,12.63 11.05,11.22 U2.2
  gndvert 0.178: v13.21,8.89 13.21,11.94 12.45,12.7 11.12,12.7 v11.05,12.63
N$20  (via drill 0.3)
  Top 0.178: R14.2 7.87,25.15 v8.38,25.65
  Bottom 0.178: CHG.1 12.93,28.19 12.06,28.19 11.43,27.56 11.43,26.8 11.18,26.54 9.27,26.54 v8.38,25.65
N$21
  Top 0.178: R18.2 15.88,15.54 Q1.1
N$22
  Top 0.178: U7.1 13.94,21.91 13.21,22.64 MEAS.4
  Bottom 0.178: MEAS.2 MEAS.4
N$23  (via drill 0.3)
  Top 0.178: v10.92,27.18 v10.91,27.19 R2.2
  Bottom 0.178: CHG_LED.1 10.55,29.08 9.66,28.19 9.66,27.18 9.92,26.92 10.79,26.92 10.92,27.05 v10.92,27.18
N$24  (via drill 0.3)
  other vias: 8.26,1.27
  pour Top (isolate 0.305): 6.35,6.35 16.51,6.35 16.51,0 6.35,0
  pour Bottom (isolate 0.305): 6.35,6.35 6.35,0 16.51,0 16.51,6.35
N$25  (via drill 0.3)
  Top 0.178: U1.15 7.93,38.68 v7.87,38.73 | U1.35 U1.34 16.4,49.51 v16.38,49.53
  gndvert 0.178: v16.38,49.53 16,49.53 14.61,48.13 14.61,41.53 14.22,41.15 v7.87,41.15
  Bottom 0.178: v7.87,38.73 7.87,39.87 | 7.87,39.87 DA_MEAS.1 | v7.87,41.15 7.87,39.87
N$26  (via drill 0.3)
  Top 0.178: U2.10 10.56,16.35 10.43,16.47 10.43,17.29 10.83,17.69 11.77,17.69 12.19,17.27 v12.19,16.76 12.19,16.74 12.06,16.6 U2.7
  pwrhorz 0.178: v19.61,11.43 13.97,11.43 13.59,11.81 13.59,16.51 13.34,16.76 v12.19,16.76
  Bottom 0.178: CH_PWR.1 v19.61,11.43
N$27  (via drill 0.3)
  other vias: 12.7,30.48
RTC_PWR_KEY  (via drill 0.3)
  Top 0.178: v6.22,49.53 6.2,49.51 U1.3 | S1.2 13.94,33.12 v13.97,33.15
  pwrhorz 0.178: v2.5,40.01 13.93,40.01 v13.97,39.97
  Bottom 0.178: J2.6 2.03,39.37 2.5,39.84 v2.5,40.01 2.5,48.35 3.68,49.53 v6.22,49.53 | v13.97,33.15 v13.97,39.97
RTC_WAKE1  (via drill 0.3)
  Top 0.178: U1.4 4.79,48.55 v3.43,48.55 | R5.2 v5.33,33.77 v5.33,33.78
  Bottom 0.178: 3.05,36.83 3.05,48.17 v3.43,48.55 | 3.05,36.83 4.83,36.83 5.33,36.32 v5.33,33.78 | 3.05,36.83 J2.7
SPI_CSB  (via drill 0.3)
  Top 0.178: v16.8,42.55 16.84,42.51 U1.27 19.73,42.51 R20.1
  pwrhorz 0.178: v8.89,45.97 2.54,45.97 1.52,46.99 J2.3
  Bottom 0.178: v16.8,42.55 9.44,42.55 8.89,43.09 v8.89,45.97
SPI_PICO  (via drill 0.3)
  Top 0.178: v19.81,40.51 U1.25
  Bottom 0.178: J2.17 20.57,41.91 19.81,41.15 v19.81,40.51
SPI_POCI  (via drill 0.3)
  Top 0.178: v19.3,39.5 18.04,39.5 U1.24
  Bottom 0.178: J2.16 20.45,44.45 19.3,43.31 v19.3,39.5
STAT_LED
  Top 0.178: J2.5 1.4,42.04 12.95,42.04 14.93,40.06 U1.22 14.93,36.24 14.04,35.35 12.11,35.35 11.67,34.91 D4.A
TCLK  (via drill 0.3)
  Top 0.178: U1.8 5.02,44.51 5.08,44.45 v6.35,44.45
  gndvert 0.178: J7.4 6.11,29.96 6.11,32.02 6.6,32.51 6.6,44.2 v6.35,44.45
TMS  (via drill 0.3)
  Top 0.178: v6.82,45.47 4.87,45.47 U1.7
  gndvert 0.178: v6.82,45.47 6.82,45.12 6.99,44.96 6.99,35.56 6.99,35.16 | J7.2 6.99,30.86 6.99,35.16 | v7.62,35.16 6.99,35.16
  Bottom 0.178: TMS.1 v7.62,35.16
U0RXI  (via drill 0.3)
  Top 0.178: U1.13 v4.83,35.06 v4.83,35.05 | v11.56,17.14 U2.8
  Bottom 0.178: v4.83,35.05 4.83,34.92 4.57,34.67 4.57,21.46 8.89,17.14 v11.56,17.14
U0TXO  (via drill 0.3)
  Top 0.178: U1.12 3.93,40.51 3.68,40.26 3.68,35.43 v4.06,35.05 | U2.9 v11.06,16.63 v11.05,16.64
  Bottom 0.178: v4.06,35.05 4.06,20.95 8.38,16.64 v11.05,16.64
U1RXI
  Top 0.178: U1.28 18.92,43.51 20.07,44.65 20.07,46.48 20.57,46.99 J2.15
U1TXO
  Top 0.178: U1.29 18.92,44.51 19.68,45.27 19.68,49.15 20.07,49.53 J2.14
V_BATT  (via drill 0.3)
  Top 0.178: 19.5,26.6 C10.1
  Top 0.305: U3.3 v18.8,26.6 19.5,26.6 | J2.12 3.3,24.13 4.06,23.37 4.06,19.43 4.71,18.78 J4.2 9.69,18.78 10.27,18.2 13.76,18.2 | Q1.3 13.76,18.2 | 13.76,18.2 17.18,18.2 18.31,19.33 18.31,22.02 v18.06,22.28
  gndvert 0.305: v18.8,26.6 18.8,25.46 18.06,24.72 v18.06,22.28
V_USB  (via drill 0.3)
  Top 0.178: R15.2 | 15.11,26.63 U3.4
  Top 0.305: C7.1 15.11,26.63 | J2.10 2.79,29.21 5.08,31.5 7.49,31.5 8.13,30.86 8.13,27.18 v8.45,26.86 8.7,26.6 U3.4 15.81,26.6 16.07,26.35 16.07,24.07 16.76,23.37 17.78,23.37 18.8,22.35 18.8,17.27 17.78,16.26 D2.A 17.78,14.6 R15.2 | R18.1 14.88,13.45 14.92,13.4 | 14.92,13.4 14.99,13.34 17.14,13.34 17.4,13.59 R15.2 | J5.VBUS1 8.98,5.36 9.17,5.17 9.17,4.67 9.78,4.06 13.08,4.06 13.69,4.67 13.69,5.17 13.88,5.36 J5.VBUS2 13.88,6.77 14.52,7.41 14.52,10.33 | D5.5 11.43,10.09 11.68,10.33 14.52,10.33 | 14.52,10.33 14.52,12.99 14.92,13.4
  Bottom 0.305: CHG_LED.2 9.51,28.83 9.26,28.57 9.26,27.67 v8.45,26.86

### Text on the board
Top: 1
gndvert: 2
pwrhorz: 3
Bottom: 4 | v10
tPlace: + | -
Measures: Units in inches
tDocu: Four Layers | Priyanka Makin

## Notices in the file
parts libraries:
SparkFun-Aesthetics: Licensing: Creative Commons ShareAlike 4.0 International - https://creativecommons.org/licenses/by-sa/4.0
SparkFun-Aesthetics: Released under the Creative Commons Attribution Share-Alike 4.0 License
SparkFun-Aesthetics: https://creativecommons.org/licenses/by-sa/4.0
